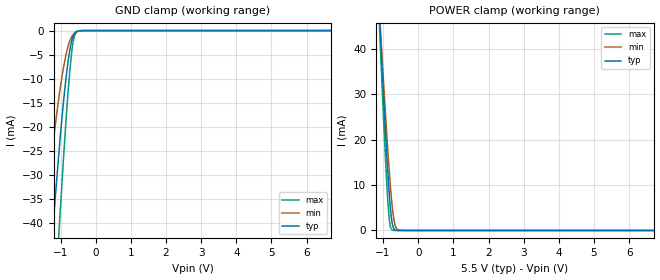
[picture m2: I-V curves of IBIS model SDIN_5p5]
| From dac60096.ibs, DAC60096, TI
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|   Model
[Model]   SDIN_5p5
Model_type   Input
Vinl = 1.5
Vinh = 3.5
|   typ   min   max
C_comp   16.3pF   16.3pF   16.3pF
[Voltage Range]   5.5   5.499   5.501
[Temperature Range]   27   105   -40
[Power Clamp Reference]   5.5   5.499   5.501
[GND Clamp Reference]   0   0   0
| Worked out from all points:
|   GND clamp passes 1 mA (typ) near -0.63 V on its own axis
|   POWER clamp passes 1 mA (typ) near -0.72 V on its own axis
[GND Clamp]
|   Voltage   I(typ)   I(min)   I(max)
-5.5V     -548.6mA   -439.5mA   -639.1mA
-1.524V   -72.71mA   -45.1mA    -103.8mA
-1.375V   -56.96mA   -34.25mA   -84.07mA
-1.26V    -45.22mA   -26.43mA   -68.96mA
-1.194V   -38.77mA   -22.25mA   -60.45mA
-1.045V   -25.17mA   -13.76mA   -41.8mA
-880mV    -12.19mA   -6.27mA    -22.5mA
-731.5mV  -3.822mA   -2.024mA   -7.923mA
-649mV    -1.306mA   -870.6uA   -2.632mA
-599.5mV  -549.1uA   -501.1uA   -1.013mA
-533.5mV  -131.4uA   -222.8uA   -211.8uA
11V       0A         0A         0A
[POWER Clamp]
|   Voltage   I(typ)   I(min)   I(max)
-5.5V     787.9mA    692.8mA    896.4mA
-1.127V   51.55mA    51.45mA    49.65mA
-1.095V   46.38mA    46.99mA    43.69mA
-1.078V   43.82mA    44.77mA    40.74mA
-929.5mV  21.64mA    25.49mA    15.57mA
-880mV    14.89mA    19.48mA    8.424mA
-847mV    10.76mA    15.68mA    4.553mA
-797.5mV  5.474mA    10.42mA    1.054mA
-731.5mV  1.232mA    4.741mA    64.9uA
-649mV    73.98uA    948.3uA    2.358uA
-451mV    0A         3.01uA     0A
11V       0A         0A         0A
